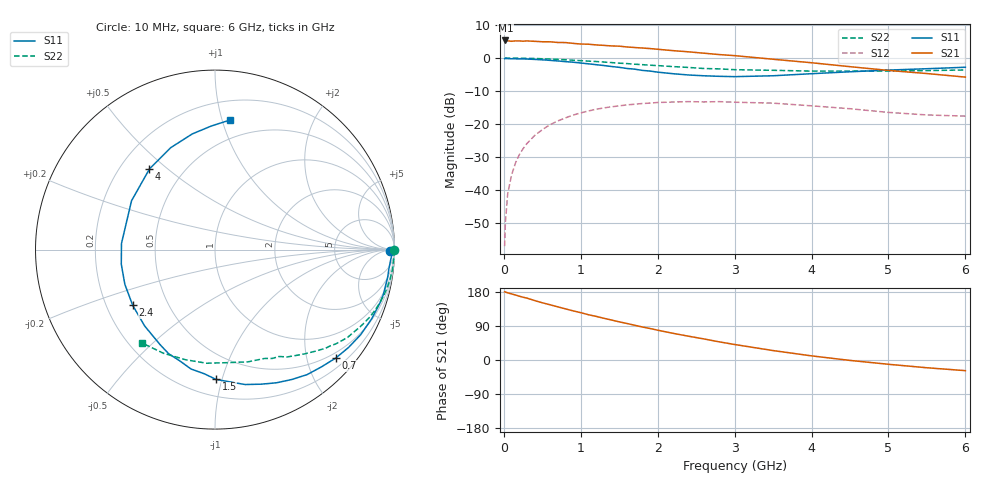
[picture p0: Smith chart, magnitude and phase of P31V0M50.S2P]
! SIEMENS Small Signal Semiconductors
! BFP181
! Si NPN RF Bipolar Junction Transistor in SOT143
! VCE = 1 V  IC = 0.5 mA
! Common Emitter S-Parameters:  March  1996
# GHz  S  MA  R  50
!  f  S11  S21  S12  S22
! GHz  MAG  ANG  MAG  ANG  MAG  ANG  MAG  ANG
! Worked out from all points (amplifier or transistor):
!   36 points, 10 MHz to 6 GHz, reference 50 ohm
!   highest |S21| = 5.3 dB at 20 MHz (marker M1)
!   |S21| within 3 dB of that: start of sweep to 2.155 GHz
!   unconditionally stable (mu >= 1): 3.593 GHz to end of sweep
!   at 250 MHz: K = 0.09, MSG = 16.3 dB, |S12| = -27.5 dB
!   at 1.4 GHz: K = 0.46, MSG = 9.2 dB, |S12| = -14.8 dB
!   at 6 GHz: K = 1.53, MAG = 1.6 dB, |S12| = -17.6 dB
!   S11 on the Smith chart (normalised r, x): 10 MHz: 70, -31; 700 MHz: 0.39, -2.56; 1.5 GHz: 0.32, -0.96; 2.4 GHz: 0.31, -0.28; 4 GHz: 0.32, +0.44; 6 GHz: 0.35, +1.06
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0.01  0.9765 -0.6  1.817 179.8  0.0014 84.7  0.9985 -0.2
0.02  0.9868 -1.3  1.849 179.5  0.0032 91.4  0.9987 -0.6
0.05  0.9814 -3.0  1.825 177.2  0.0087 90.6  0.9979 -1.5
0.1  0.9749 -6.2  1.797 174.4  0.0167 84.9  0.9969 -3.0
0.15  0.9742 -9.2  1.822 171.5  0.0254 83.7  0.9952 -4.5
0.2  0.9713 -12.0  1.818 168.5  0.034 81.3  0.9957 -6.1
0.3  0.9655 -18.1  1.819 163.3  0.0504 76.9  0.9902 -9.1
0.4  0.9541 -23.9  1.794 156.9  0.0668 73.0  0.9843 -12.0
0.6  0.9226 -36.2  1.764 145.8  0.0974 64.5  0.9653 -17.8
0.7  0.9043 -41.9  1.723 140.3  0.111 60.3  0.9536 -20.7
0.8  0.8824 -47.8  1.717 135.0  0.1236 56.2  0.942 -23.3
1.1  0.8174 -65.2  1.622 119.5  0.1574 44.9  0.8989 -30.8
1.5  0.723 -89.6  1.515 100.7  0.1882 31.4  0.8364 -39.9
1.9  0.635 -114.0  1.393 83.1  0.2075 19.7  0.7789 -47.5
2.2  0.5784 -132.7  1.295 70.4  0.2151 12.0  0.7419 -52.7
2.4  0.5537 -145.9  1.243 62.8  0.2182 7.1  0.7205 -56.1
3  0.5222 176.3  1.088 40.9  0.2138 -5.5  0.6661 -65.6
3.5  0.5387 149.7  0.959 24.9  0.2069 -13.5  0.6517 -73.7
4  0.5789 129.1  0.849 10.9  0.1885 -20.1  0.6339 -83.5
4.5  0.6191 113.5  0.74 -1.1  0.1703 -25.5  0.6348 -94.2
5.5  0.6889 91.7  0.582 -20.5  0.137 -23.7  0.645 -116.4
6  0.7256 83.6  0.514 -28.1  0.1315 -20.0  0.6599 -127.9
